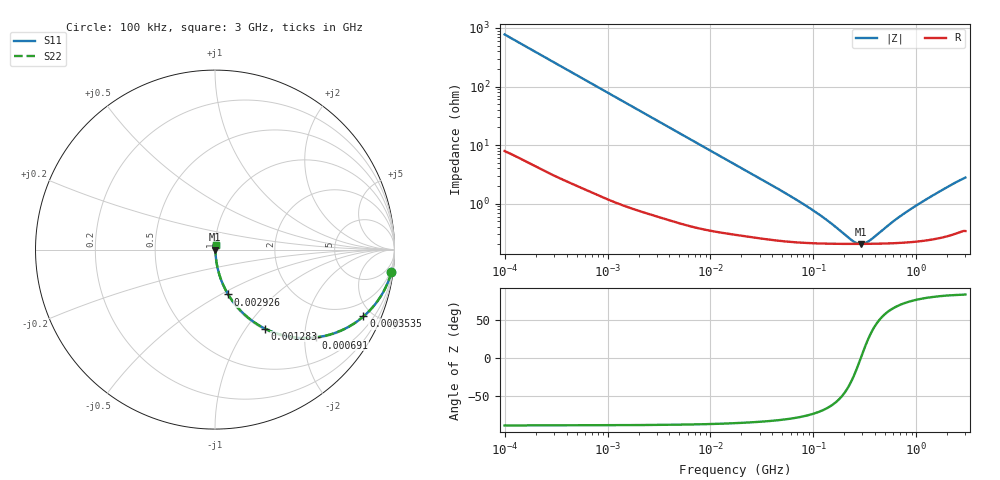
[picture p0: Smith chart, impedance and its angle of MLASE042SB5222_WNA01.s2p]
! MLASE042SB5222_WNA01  S-PARAMETER MODEL  ( Standard Model )
! Model Generated by TAIYO YUDEN Corporation (http://www.ty-top.com)
! Version 1.0
! TAIYO YUDEN Control No. 220601
! Copyright(c) 2016 TAIYO YUDEN CO.,LTD. All Rights Reserved.
! Product Description (link to TY-COMPAS)
! https://ds.yuden.co.jp/TYCOMPAS/or/detail?pn=MLASE042SB5222KWNA01&u=M
! Products Name : Multilayer Ceramic Capacitors
! Characteristics :
!  Capacitance : 2200 [pF] , Rated Voltage : 16 [V] , TCC : X5R
!  Case Size : 0.4 x 0.2 / 0.016 x 0.008 [mm/inch] , Thickness : 0.2 / 0.008 [mm/inch]
!  (Conditions: Temperature = 25 [degC] , DC Bias Voltage = 0 [V])
! External Node Assignments :
!  1  o---| |---o  2
! GND o---------o GND
! Frequency Range : 100kHz  -  3GHz  [ 401 STEP ]
# MHZ S RI R 50
! Freq[MHz].  S11 Real  S11 Imag  S21 Real  S21 Imag  S12 Real  S12 Imag  S22 Real  S22 Imag
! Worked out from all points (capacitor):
!   401 points, 100 kHz to 3 GHz, reference 50 ohm
!   read as one part in series: C = 2.05 nF near 105.3 kHz
!   lowest |Z| = 205 mohm at 287.5 MHz (marker M1)
!   series resonance near 290 MHz, so ESL is about 150 pH
!   S11 on the Smith chart (normalised r, x): 100 kHz: 1, -15; 353.5 kHz: 1.05, -4.42; 691 kHz: 1.03, -2.27; 1.283 MHz: 1.02, -1.23; 2.926 MHz: 1.01, -0.54; 3 GHz: 1.01, +0.06
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0.1  0.9824 -0.1266  0.0176 0.1266  0.0176 0.1266  0.9824 -0.1266
0.205778  0.9324 -0.2455  0.0676 0.2455  0.0676 0.2455  0.9324 -0.2455
0.353547  0.8273 -0.3721  0.1727 0.3721  0.1727 0.3721  0.8273 -0.3721
0.562235  0.6587 -0.4676  0.3413 0.4676  0.3413 0.4676  0.6587 -0.4676
0.690972  0.563 -0.4892  0.437 0.4892  0.437 0.4892  0.563 -0.4892
0.917447  0.4252 -0.4871  0.5748 0.4871  0.5748 0.4871  0.4252 -0.4871
1.282589  0.2779 -0.44  0.7221 0.44  0.7221 0.44  0.2779 -0.44
1.887902  0.1541 -0.3519  0.8459 0.3519  0.8459 0.3519  0.1541 -0.3519
2.925885  0.0736 -0.2501  0.9264 0.2501  0.9264 0.2501  0.0736 -0.2501
3.161081  0.0644 -0.234  0.9356 0.234  0.9356 0.234  0.0644 -0.234
6.848882  0.0173 -0.1145  0.9827 0.1145  0.9827 0.1145  0.0173 -0.1145
17.7727  0.00494 -0.0451  0.9951 0.0451  0.9951 0.0451  0.00494 -0.0451
51.12795  0.00251 -0.0156  0.9975 0.0156  0.9975 0.0156  0.00251 -0.0156
97.38194  0.00215 -0.00752  0.9978 0.00752  0.9978 0.00752  0.00215 -0.00752
143.341  0.00207 -0.00436  0.9979 0.00436  0.9979 0.00436  0.00207 -0.00436
233.9019  0.00204 -0.00124  0.998 0.00124  0.998 0.00124  0.00204 -0.00124
287.4592  0.00204 -5e-05  0.998 5e-05  0.998 5e-05  0.00204 -5e-05
353.2796  0.00205 0.00113  0.998 -0.00113  0.998 -0.00113  0.00205 0.00113
547.5153  0.0021 0.00387  0.9979 -0.00387  0.9979 -0.00387  0.0021 0.00387
1186.261  0.00243 0.0109  0.9976 -0.0109  0.9976 -0.0109  0.00243 0.0109
2259.438  0.00338 0.0212  0.9966 -0.0212  0.9966 -0.0212  0.00338 0.0212
3000  0.00413 0.0273  0.9959 -0.0273  0.9959 -0.0273  0.00413 0.0273
